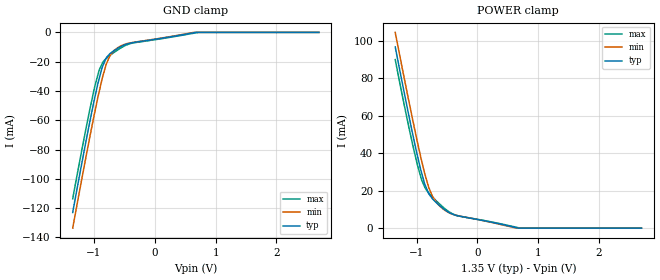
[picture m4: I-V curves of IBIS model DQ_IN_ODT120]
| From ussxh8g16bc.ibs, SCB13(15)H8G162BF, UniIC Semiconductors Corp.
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| MODEL DQ_IN_ODT120 (Data Input with 120ohm ODT, 800-2133Mbps)
[Model]   DQ_IN_ODT120
Model_type   Input
Vinl = 545.000mV
Vinh = 805.000mV
|   typ   min   max
|C_comp   0.948pF   0.899pF   0.999pF
C_comp_power_clamp   0.4740pF   0.4495pF   0.4995pF
C_comp_gnd_clamp   0.4740pF   0.4495pF   0.4995pF
| Note: C_comp changes when the ODT circuit is enabled.
[Model Spec]
| Input threshold voltage corners
Vinl   0.5450V   0.5115V   0.5825V
Vinh   0.8050V   0.7715V   0.8425V
| Dynamic Overshoot Parameters from DDR3L Specification
|D_overshoot_ampl_h   0.40   NA   NA
|D_overshoot_ampl_l   0.40   NA   NA
|D_overshoot_area_h   0.11n   NA   NA
|D_overshoot_area_l   0.11n   NA   NA
[Receiver Thresholds]
Vth   =  0.675V
Vth_min  =  0.6615V
Vth_max  =  0.6885V
Vinh_ac  =  0.130V
Vinh_dc  =  0.090V
Vinl_ac  = -0.130V
Vinl_dc  = -0.090V
Tslew_ac =  5.000ns |Not specified, so set to high value
Threshold_sensitivity = 0.50
Reference_supply Power_clamp_ref
[Voltage Range]   1.3500V   1.2830V   1.4250V
[POWER Clamp Reference]   1.3500V   1.2830V   1.4250V
| Junction Temperature (Ambient temp is 40C typ, 85C min, 0C max)
[Temperature Range]   45.0   90.0   0.0
[GND Clamp]
|   Voltage   I(typ)   I(min)   I(max)
-1.35V    -122.9mA   -133.6mA   -113.6mA
-1.195V   -88.01mA   -98.7mA    -79.04mA
-1.055V   -58.03mA   -68.41mA   -49.75mA
-985mV    -44.04mA   -53.96mA   -36.49mA
-915mV    -31.52mA   -40.39mA   -25.7mA
-870mV    -24.43mA   -32.23mA   -21.67mA
-800mV    -17.42mA   -21.76mA   -17.84mA
-730mV    -14.25mA   -15.3mA    -15.51mA
-665mV    -12.32mA   -12.16mA   -13.54mA
-405mV    -7.395mA   -7.167mA   -7.689mA
720mV     0A         0A         0A
2.7V      0A         0A         0A
[POWER Clamp]
|   Voltage   I(typ)   I(min)   I(max)
-1.35V    96.85mA    104.6mA    90.03mA
-1.195V   71.14mA    78.95mA    64.63mA
-1.055V   48.99mA    56.61mA    43.33mA
-985mV    38.64mA    45.92mA    33.69mA
-915mV    29.32mA    35.84mA    25.66mA
-870mV    24.01mA    29.74mA    22.36mA
-800mV    18.43mA    21.79mA    18.85mA
-735mV    15.56mA    16.79mA    16.55mA
-560mV    10.44mA    10.15mA    11.08mA
-340mV    6.726mA    6.783mA    6.776mA
705mV     0A         0A         0A
2.7V      0A         0A         0A
